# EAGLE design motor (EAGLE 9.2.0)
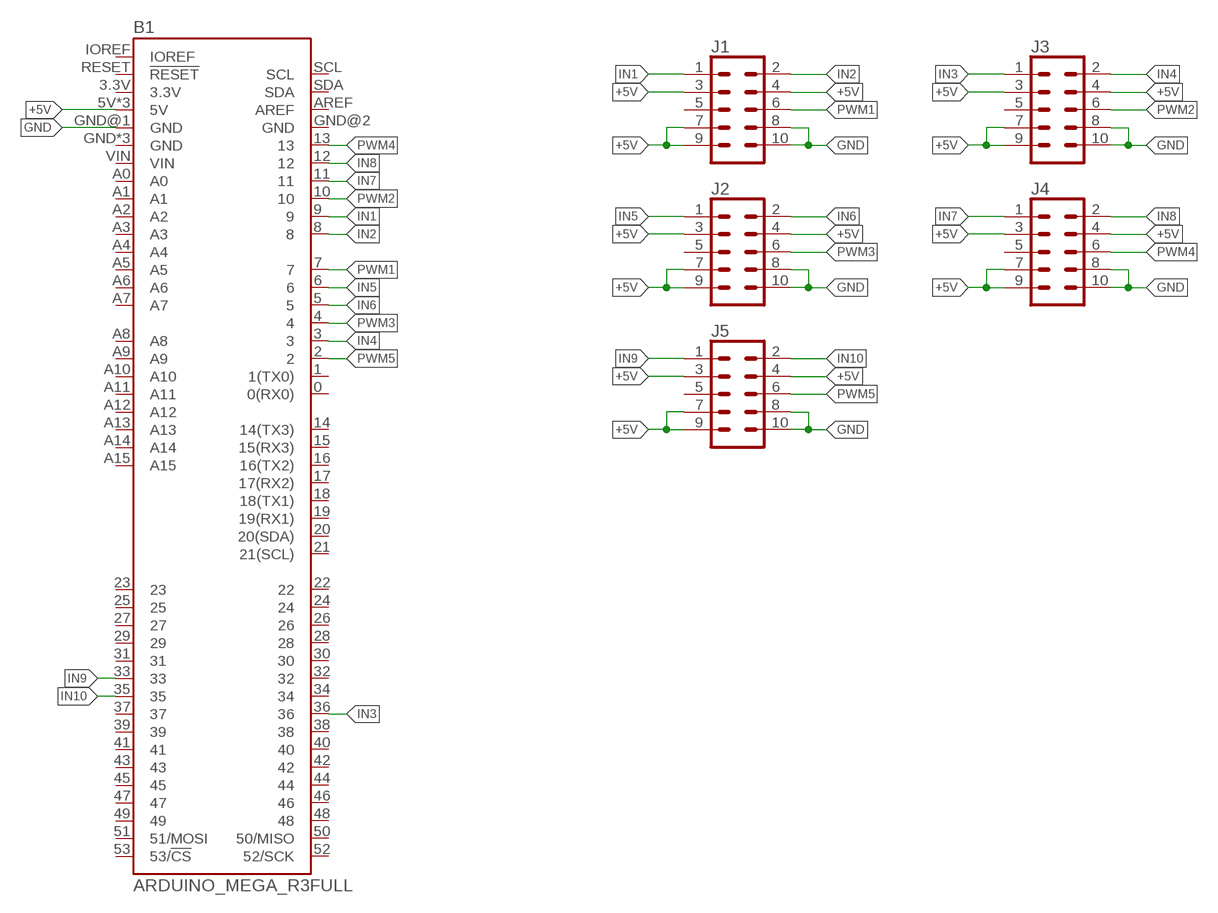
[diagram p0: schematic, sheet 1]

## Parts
B1  ARDUINO_MEGA_R3FULL  [ARDUINO_MEGA_NO_SILK]
J1  CONN_05X2SHD-NS  [2X5-SHROUDED-NS]
J2  CONN_05X2SHD-NS  [2X5-SHROUDED-NS]
J3  CONN_05X2SHD-NS  [2X5-SHROUDED-NS]
J4  CONN_05X2SHD-NS  [2X5-SHROUDED-NS]
J5  CONN_05X2SHD-NS  [2X5-SHROUDED-NS]

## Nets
+5V: B1.5V B1.5V@1(5V) B1.5V@2(5V) J1.3 J1.4 J1.7 J1.9 J2.3 J2.4 J2.7 J2.9 J3.3 J3.4 J3.7 J3.9 J4.3 J4.4 J4.7 J4.9 J5.3 J5.4 J5.7 J5.9
GND: B1.GND@1(GND) J1.8 J1.10 J2.8 J2.10 J3.8 J3.10 J4.8 J4.10 J5.8 J5.10
IN1: B1.9 J1.1
IN2: B1.8 J1.2
IN3: B1.36 J3.1
IN4: B1.3 J3.2
IN5: B1.6 J2.1
IN6: B1.5 J2.2
IN7: B1.11 J4.1
IN8: B1.12 J4.2
IN9: B1.33 J5.1
IN10: B1.35 J5.2
PWM1: B1.7 J1.6
PWM2: B1.10 J3.6
PWM3: B1.4 J2.6
PWM4: B1.13 J4.6
PWM5: B1.2 J5.6
Unconnected: B1.0(0(RX0)) B1.1(1(TX0)) B1.3.3V B1.14(14(TX3)) B1.15(15(RX3)) B1.16(16(TX2)) B1.17(17(RX2)) B1.18(18(TX1)) B1.19(19(RX1)) B1.20(20(SDA)) B1.21(21(SCL)) B1.22 B1.23 B1.24 B1.25 B1.26 B1.27 B1.28 B1.29 B1.30 B1.31 B1.32 B1.34 B1.37 B1.38 B1.39 B1.40 B1.41 B1.42 B1.43 B1.44 B1.45 B1.46 B1.47 B1.48 B1.49 B1.50(50/MISO) B1.51(51/MOSI) B1.52(52/SCK) B1.53(53/!CS) B1.A0 B1.A1 B1.A2 B1.A3 B1.A4 B1.A5 B1.A6 B1.A7 B1.A8 B1.A9 B1.A10 B1.A11 B1.A12 B1.A13 B1.A14 B1.A15 B1.AREF B1.GND B1.GND@2(GND) B1.GND@3(GND) B1.GND@4(GND) B1.IOREF B1.RESET(!RESET) B1.SCL B1.SDA B1.VIN J1.5 J2.5 J3.5 J4.5 J5.5

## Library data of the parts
B1 = SparkFun-Boards:ARDUINO_MEGA_R3: Arduino Mega R3 ATmega2560 R3 compatible footprint. SparkFun Products: Arduino Mega 2560 R3
J1-J5 = SparkFun-Connectors:CONN_05X2: Multi connection point. Often used as Generic Header-pin footprint for 0.1 inch spaced/style header connections For AVR SPI programming port, see special device with nice symbol: "AVR_SPI_PROG_5x2.dev" You can populate with any combo of single row headers, but if you'd like an exact match, check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; PROD_ID: CONN-08671; SF_ID: PRT-08506

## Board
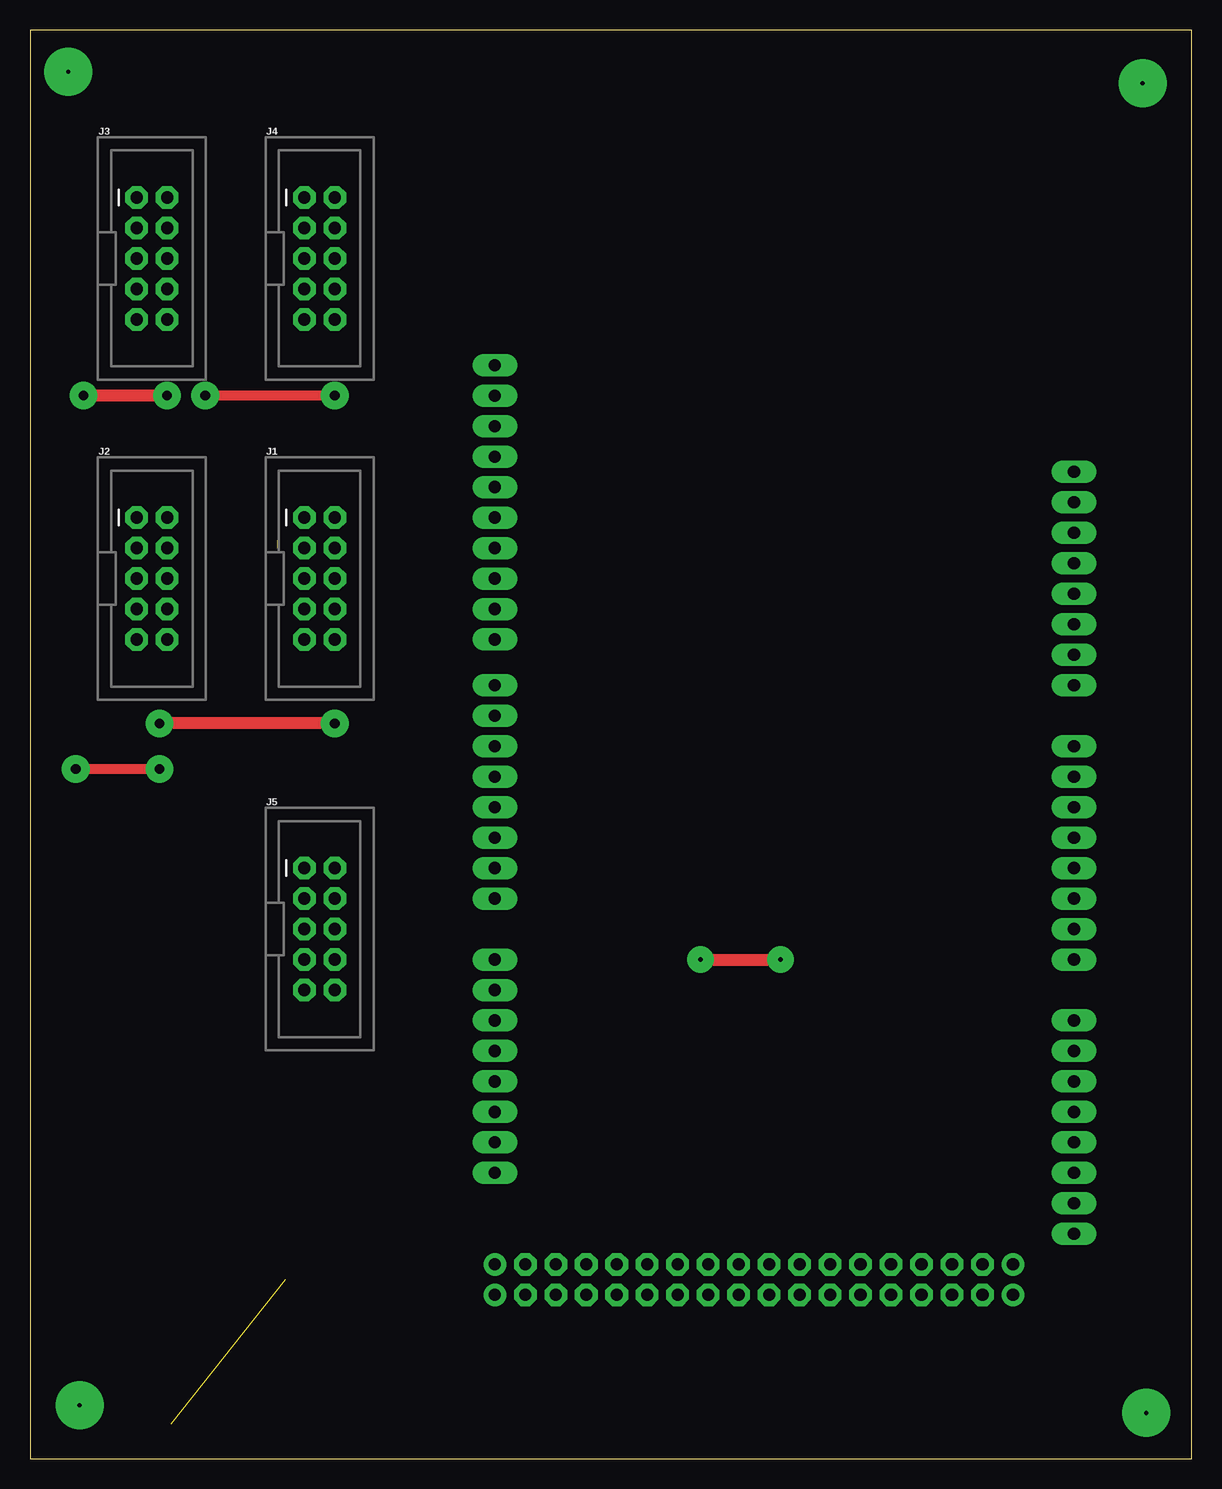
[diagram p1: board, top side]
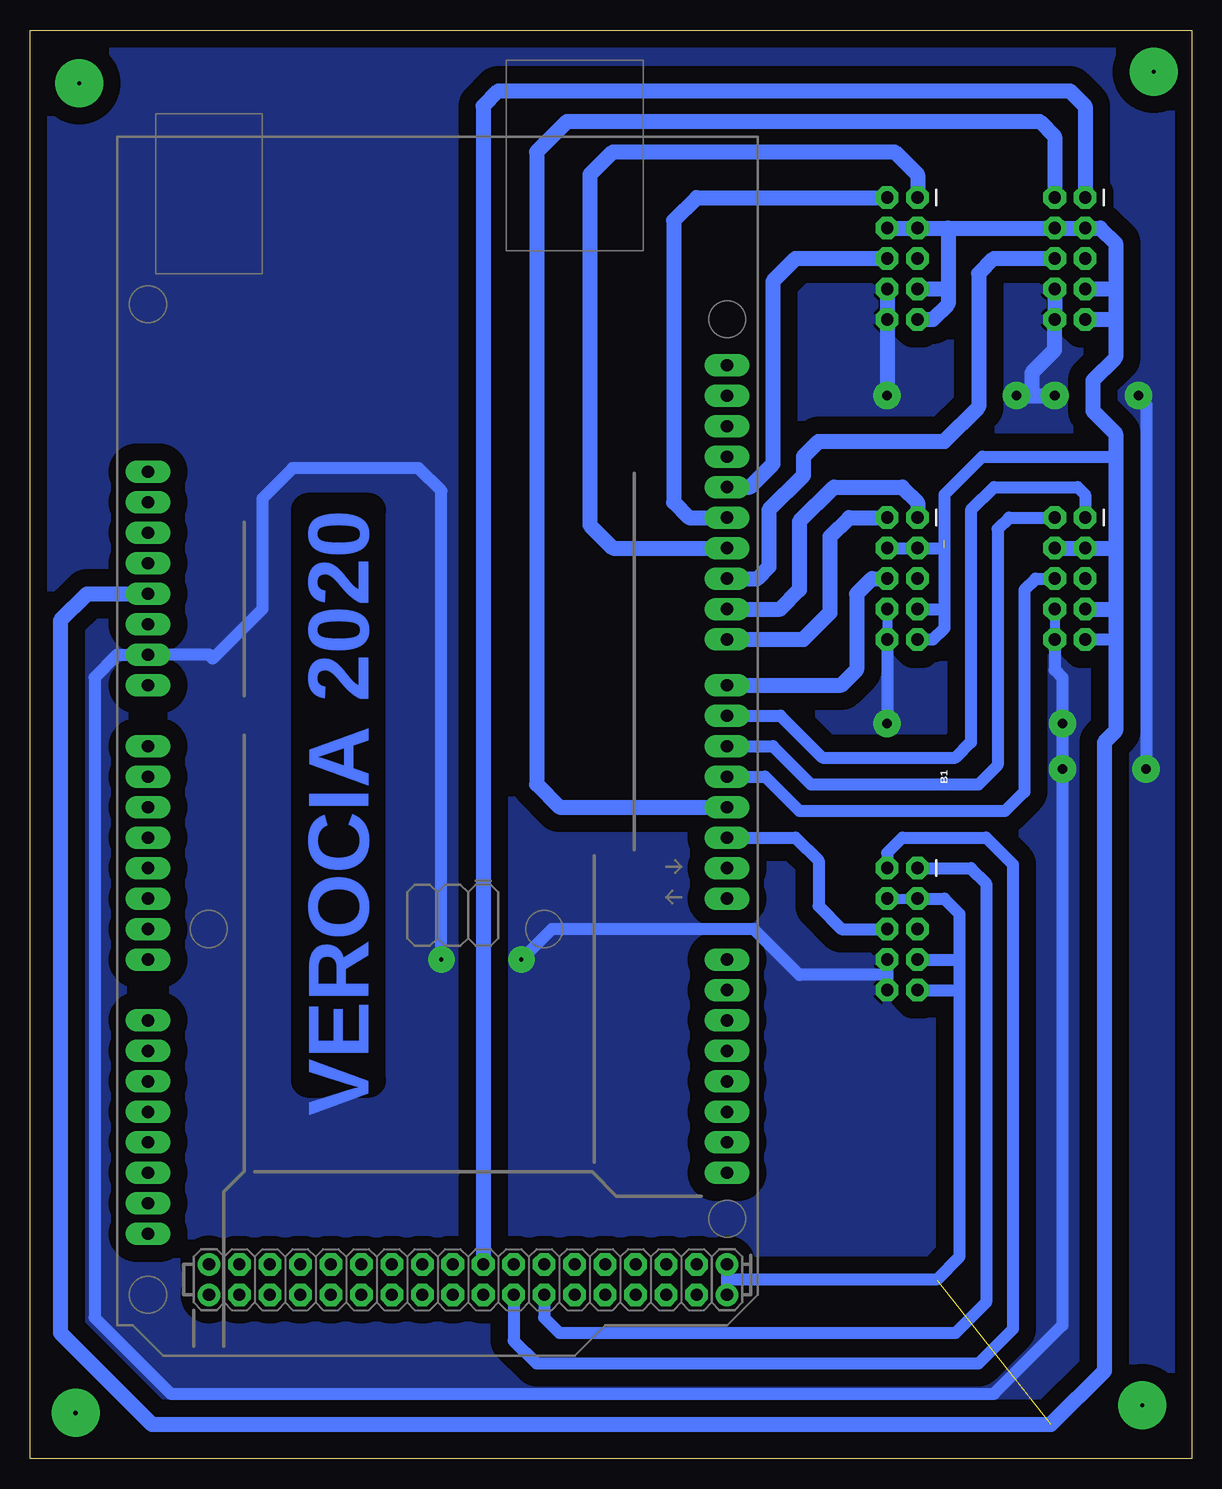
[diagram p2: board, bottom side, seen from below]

Size 96.83 x 119.05 mm. Coordinates in mm from the lower left corner, seen from the top.
Outline: 0,0 96.83,0 96.83,119.05 0,119.05 0,0
Copper layers (1*16): Top 0.035mm / dielectric 1.5mm / Bottom 0.035mm
Design rules "default": minimum track width 6mil, minimum drill 0.35mm, track to track 6mil, track to pad 6mil, pad to pad 6mil, via to via 6mil, smd to smd 6mil, copper to edge 40mil, drill to drill 6mil, minimum pad ring 10mil, minimum via ring 8mil, stop-mask expansion 4mil, vias tented up to drill 0mil, thermal gap 10mil

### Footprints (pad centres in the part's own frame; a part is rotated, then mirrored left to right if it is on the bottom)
ARDUINO_MEGA_NO_SILK = drill 1.016 pad 1.88 long: 0 13.97,24.13; 1 11.43,24.13; 2 8.89,24.13; 3 6.35,24.13; 3.3V -13.97,-24.13; 4 3.81,24.13; 5 1.27,24.13; 5V -11.43,-24.13; 6 -1.27,24.13; 7 -3.81,24.13; 8 -7.62,24.13; 9 -10.16,24.13; 10 -12.7,24.13; 11 -15.24,24.13; 12 -17.78,24.13; 13 -20.32,24.13; 14 19.05,24.13; 15 21.59,24.13; 16 24.13,24.13; 17 26.67,24.13; 18 29.21,24.13; 19 31.75,24.13; 20 34.29,24.13; 21 36.83,24.13; A0 1.27,-24.13; A1 3.81,-24.13; A2 6.35,-24.13; A3 8.89,-24.13; A4 11.43,-24.13; A5 13.97,-24.13; A6 16.51,-24.13; A7 19.05,-24.13; A8 24.13,-24.13; A9 26.67,-24.13; A10 29.21,-24.13; A11 31.75,-24.13; A12 34.29,-24.13; A13 36.83,-24.13; A14 39.37,-24.13; A15 41.91,-24.13; AREF -25.4,24.13; GND -8.89,-24.13; GND@1 -6.35,-24.13; GND@4 -22.86,24.13; IOREF -19.05,-24.13; NC -21.59,-24.13; RESET -16.51,-24.13; SCL -30.48,24.13; SDA -27.94,24.13; VIN -3.81,-24.13 | drill 1.016 pad 1.88: 5V@1 44.45,24.13; 5V@2 46.99,24.13; GND@2 44.45,-19.05; GND@3 46.99,-19.05 | drill 1.016 pad 1.88 octagon: 22 44.45,21.59; 23 46.99,21.59; 24 44.45,19.05; 25 46.99,19.05; 26 44.45,16.51; 27 46.99,16.51; 28 44.45,13.97; 29 46.99,13.97; 30 44.45,11.43; 31 46.99,11.43; 32 44.45,8.89; 33 46.99,8.89; 34 44.45,6.35; 35 46.99,6.35; 36 44.45,3.81; 37 46.99,3.81; 38 44.45,1.27; 39 46.99,1.27; 40 44.45,-1.27; 41 46.99,-1.27; 42 44.45,-3.81; 43 46.99,-3.81; 44 44.45,-6.35; 45 46.99,-6.35; 46 44.45,-8.89; 47 46.99,-8.89; 48 44.45,-11.43; 49 46.99,-11.43; 50 44.45,-13.97; 51 46.99,-13.97; 52 44.45,-16.51; 53 46.99,-16.51
2X5-SHROUDED-NS = drill 1.016 pad 1.88 octagon: 1 -1.27,5.08; 2 1.27,5.08; 3 -1.27,2.54; 4 1.27,2.54; 5 -1.27,0; 6 1.27,0; 7 -1.27,-2.54; 8 1.27,-2.54; 9 -1.27,-5.08; 10 1.27,-5.08

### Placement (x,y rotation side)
B1  62.87,60.64 270 bottom
J1  24.13,73.34 0 top
J2  10.16,73.34 0 top
J3  10.16,100.01 0 top
J4  24.13,100.01 0 top
J5  24.13,44.13 0 top

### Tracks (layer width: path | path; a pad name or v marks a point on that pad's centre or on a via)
+5V  (2 unrouted)
  Bottom 0.813: J2.3 6.99,75.88 | J5.4 J5.3 | J4.3 20.32,102.55
  Bottom 1.016: J1.4 J1.3 20.64,75.88 20.64,80.33 17.46,83.5 6.35,83.5 | 20.64,76.52 20.64,70.8 | 20.64,70.8 20.64,69.22 21.59,68.26 J1.9 | J1.7 20.64,70.8 | J2.9 6.35,68.26 | B1.5V@2 38.73,14.92 | 38.73,14.92 B1.5V@1 | 38.73,14.92 21.27,14.92 19.37,16.83 19.37,39.05 | J5.3 20.64,46.67 19.37,45.4 19.37,41.59 | 19.37,41.59 19.37,39.05 | J5.9 19.37,39.05 | J5.7 19.37,41.59
  Bottom 1.27: J2.4 J2.3 6.35,75.88 | J4.9 21.59,94.93 20.32,96.2 20.32,97.47 | 20.32,102.55 20.32,97.47 | J4.4 J4.3 J3.4 J3.3 7.62,102.55 6.35,101.28 6.35,97.47 | J4.7 20.32,97.47 | 6.35,70.8 6.35,68.26 6.35,60.64 7.3,59.69 7.3,7.3 11.75,2.86 86.68,2.86 94.3,10.48 94.3,69.85 92.08,72.07 B1.5V | J2.7 6.35,70.8 | 6.35,75.88 6.35,70.8 | 6.35,75.88 6.35,83.5 6.35,85.41 8.26,87.31 8.26,89.85 6.35,91.76 6.35,94.93 | 6.35,97.47 6.35,94.93 | J3.7 6.35,97.47 | J3.9 6.35,94.93
GND  (via drill 0.35 pad 2.2, 0.8 pad 2.3)
  Top 0.813: v25.4,88.58 v14.61,88.58 | v10.79,57.47 v3.81,57.47
  Top 1.016: v11.43,88.58 v4.45,88.58 | v25.4,61.28 v10.79,61.28 | v55.88,41.59 v62.55,41.59
  Bottom 0.813: J2.8 J2.10 | v14.61,88.58 13.34,88.58 | J1.8 J1.10
  Bottom 1.016: J5.8 25.4,40.32 | 25.4,40.32 J5.10 | J2.10 11.43,65.72 10.79,65.09 v10.79,61.28 v10.79,57.47 10.79,11.11 16.51,5.4 85.09,5.4 91.44,11.75 91.44,65.09 89.53,66.99 B1.GND@1 | v4.45,88.58 3.81,87.95 v3.81,57.47 | J1.10 v25.4,61.28 | 86.36,66.99 B1.GND@1 | v62.55,41.59 62.55,80.64 64.45,82.55 74.93,82.55 77.47,80.01 77.47,70.8 81.6,66.68 81.92,66.99 B1.GND@1 | 25.4,40.32 32.7,40.32 36.51,44.13 53.34,44.13 v55.88,41.59
  Bottom 1.27: J4.8 J4.10 v25.4,88.58 | J3.8 J3.10 11.43,92.39 13.34,90.49 13.34,88.58 | v14.61,88.58 v11.43,88.58
  pour Bottom (isolate 1.422): 0,0 0,119.06 96.84,119.06 96.84,0
IN1
  Bottom 1.27: J1.1 22.86,79.69 24.13,80.96 29.84,80.96 32.7,78.11 32.7,72.39 34.29,70.8 B1.9
IN2
  Bottom 1.27: J1.2 28.57,78.42 30.16,76.84 30.16,70.48 32.38,68.26 B1.8
IN3
  Bottom 1.27: J3.1 8.89,112.71 10.16,113.98 57.78,113.98 59.05,112.71 B1.36
IN4
  Bottom 1.27: J3.2 11.43,110.17 12.7,111.44 52.07,111.44 54.61,108.9 54.61,56.2 52.7,54.29 B1.3
IN5
  Bottom 1.016: J2.1 8.89,80.33 9.53,80.96 16.51,80.96 18.41,79.06 18.41,59.69 19.68,58.42 30.8,58.42 34.29,61.91 B1.6
IN6
  Bottom 1.016: J2.2 15.24,78.42 16.19,77.47 16.19,57.79 17.78,56.2 31.75,56.2 34.92,59.37 B1.5
IN7
  Bottom 1.27: B1.11 48.26,75.88 50.16,77.79 50.16,107 48.26,108.9 24.77,108.9 22.86,107 J4.1
IN8
  Bottom 1.27: B1.12 41.91,78.42 43.18,79.69 43.18,103.19 41.27,105.09 J4.2
IN9
  Bottom 1.016: J5.1 18.41,49.21 17.14,47.94 17.14,13.02 19.68,10.48 52.7,10.48 53.98,11.75 B1.33
IN10
  Bottom 1.016: J5.2 25.4,50.48 24.13,51.75 17.14,51.75 14.92,49.53 14.92,10.8 17.78,7.94 54.61,7.94 56.52,9.84 B1.35
N$3  (via drill 0.35 pad 4)
  other vias: 3.17,115.57
N$4  (via drill 0.35 pad 4)
  other vias: 92.71,114.62
N$5  (via drill 0.35 pad 4)
  other vias: 93.03,3.81
N$6  (via drill 0.35 pad 4)
  other vias: 4.13,4.45
PWM1
  Bottom 1.27: J1.6 26.67,73.34 27.94,72.07 27.94,65.72 29.21,64.45 B1.7
PWM2
  Bottom 1.27: J3.6 16.51,100.01 17.78,98.74 17.78,87.63 20.64,84.77 31.11,84.77 32.38,83.5 32.38,81.92 35.24,79.06 35.24,74.3 36.2,73.34 B1.10
PWM3
  Bottom 1.016: J2.6 13.02,73.34 13.97,72.39 13.97,55.56 15.56,53.97 32.7,53.97 35.56,56.83 B1.4
PWM4
  Bottom 1.27: J4.6 33.02,100.01 34.92,98.11 34.92,82.87 36.83,80.96 B1.13
PWM5
  Bottom 1.016: J5.6 29.21,44.13 31.11,46.04 31.11,49.85 33.02,51.75 B1.2

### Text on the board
Bottom: VEROCIA 2020

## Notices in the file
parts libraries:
SparkFun-Connectors: Licensing: Creative Commons ShareAlike 4.0 International - https://creativecommons.org/licenses/by-sa/4.0
